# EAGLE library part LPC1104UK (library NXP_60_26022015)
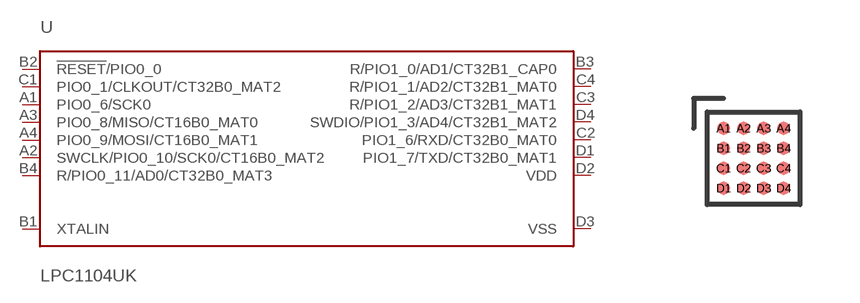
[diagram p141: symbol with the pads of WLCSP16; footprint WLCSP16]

Designator prefix U

## LPC1104UK  [WLCSP16]
A1  PIO0_6/SCK0
A2  SWCLK/PIO0_10/SCK0/CT16B0_MAT2
A3  PIO0_8/MISO/CT16B0_MAT0
A4  PIO0_9/MOSI/CT16B0_MAT1
B1  XTALIN  in
B2  !RESET!/PIO0_0
B3  R/PIO1_0/AD1/CT32B1_CAP0
B4  R/PIO0_11/AD0/CT32B0_MAT3
C1  PIO0_1/CLKOUT/CT32B0_MAT2
C2  PIO1_6/RXD/CT32B0_MAT0
C3  R/PIO1_2/AD3/CT32B1_MAT1
C4  R/PIO1_1/AD2/CT32B1_MAT0
D1  PIO1_7/TXD/CT32B0_MAT1
D2  VDD  pwr
D3  VSS  pwr
D4  SWDIO/PIO1_3/AD4/CT32B1_MAT2

## Footprint WLCSP16 (pad centres in mm)
WLCSP16 - Wafer Level Chip-Size Package LPC1102UK PLEASE DO NOT USE
smd 0.32 x 0.32: A1 -0.75,0.75; A2 -0.25,0.75; A3 0.25,0.75; A4 0.75,0.75; B1 -0.75,0.25; B2 -0.25,0.25; B3 0.25,0.25; B4 0.75,0.25; C1 -0.75,-0.25; C2 -0.25,-0.25; C3 0.25,-0.25; C4 0.75,-0.25; D1 -0.75,-0.75; D2 -0.25,-0.75; D3 0.25,-0.75; D4 0.75,-0.75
